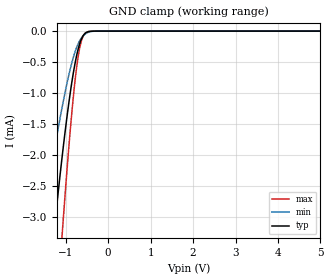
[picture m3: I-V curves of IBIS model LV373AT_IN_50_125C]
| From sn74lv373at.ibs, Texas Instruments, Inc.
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[Model]   LV373AT_IN_50_125C
Model_type  Input
Vinl=0.8
Vinh=2.0
| variable   typ   min   max
C_comp   4pF   NA   10pF
[Temperature Range]   40   140   -40
| Ambient temperature   25   125   -40
[Voltage range]   5   4.5   5.5
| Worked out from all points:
|   GND clamp passes 1 mA (typ) near -0.89 V on its own axis
[GND Clamp]
| LV373AT_IN_50
|   Voltage   I(typ)   I(min)   I(max)
-5V       -39.32mA   -23.19mA   -50.37mA
-1.595V   -5.577mA   -3.328mA   -8.605mA
-1.54V    -5.154mA   -3.08mA    -7.998mA
-1.28V    -3.276mA   -1.973mA   -5.225mA
-1.25V    -3.075mA   -1.853mA   -4.918mA
-1.08V    -2.002mA   -1.212mA   -3.244mA
-885mV    -959.1uA   -589.6uA   -1.541mA
-745mV    -403.2uA   -268.4uA   -599.7uA
-690mV    -248.8uA   -181.1uA   -344.9uA
-630mV    -128.1uA   -111.1uA   -159.3uA
-495mV    -16.08uA   -27.93uA   -13.87uA
5V        17.64nA    5.869nA    163.4nA
